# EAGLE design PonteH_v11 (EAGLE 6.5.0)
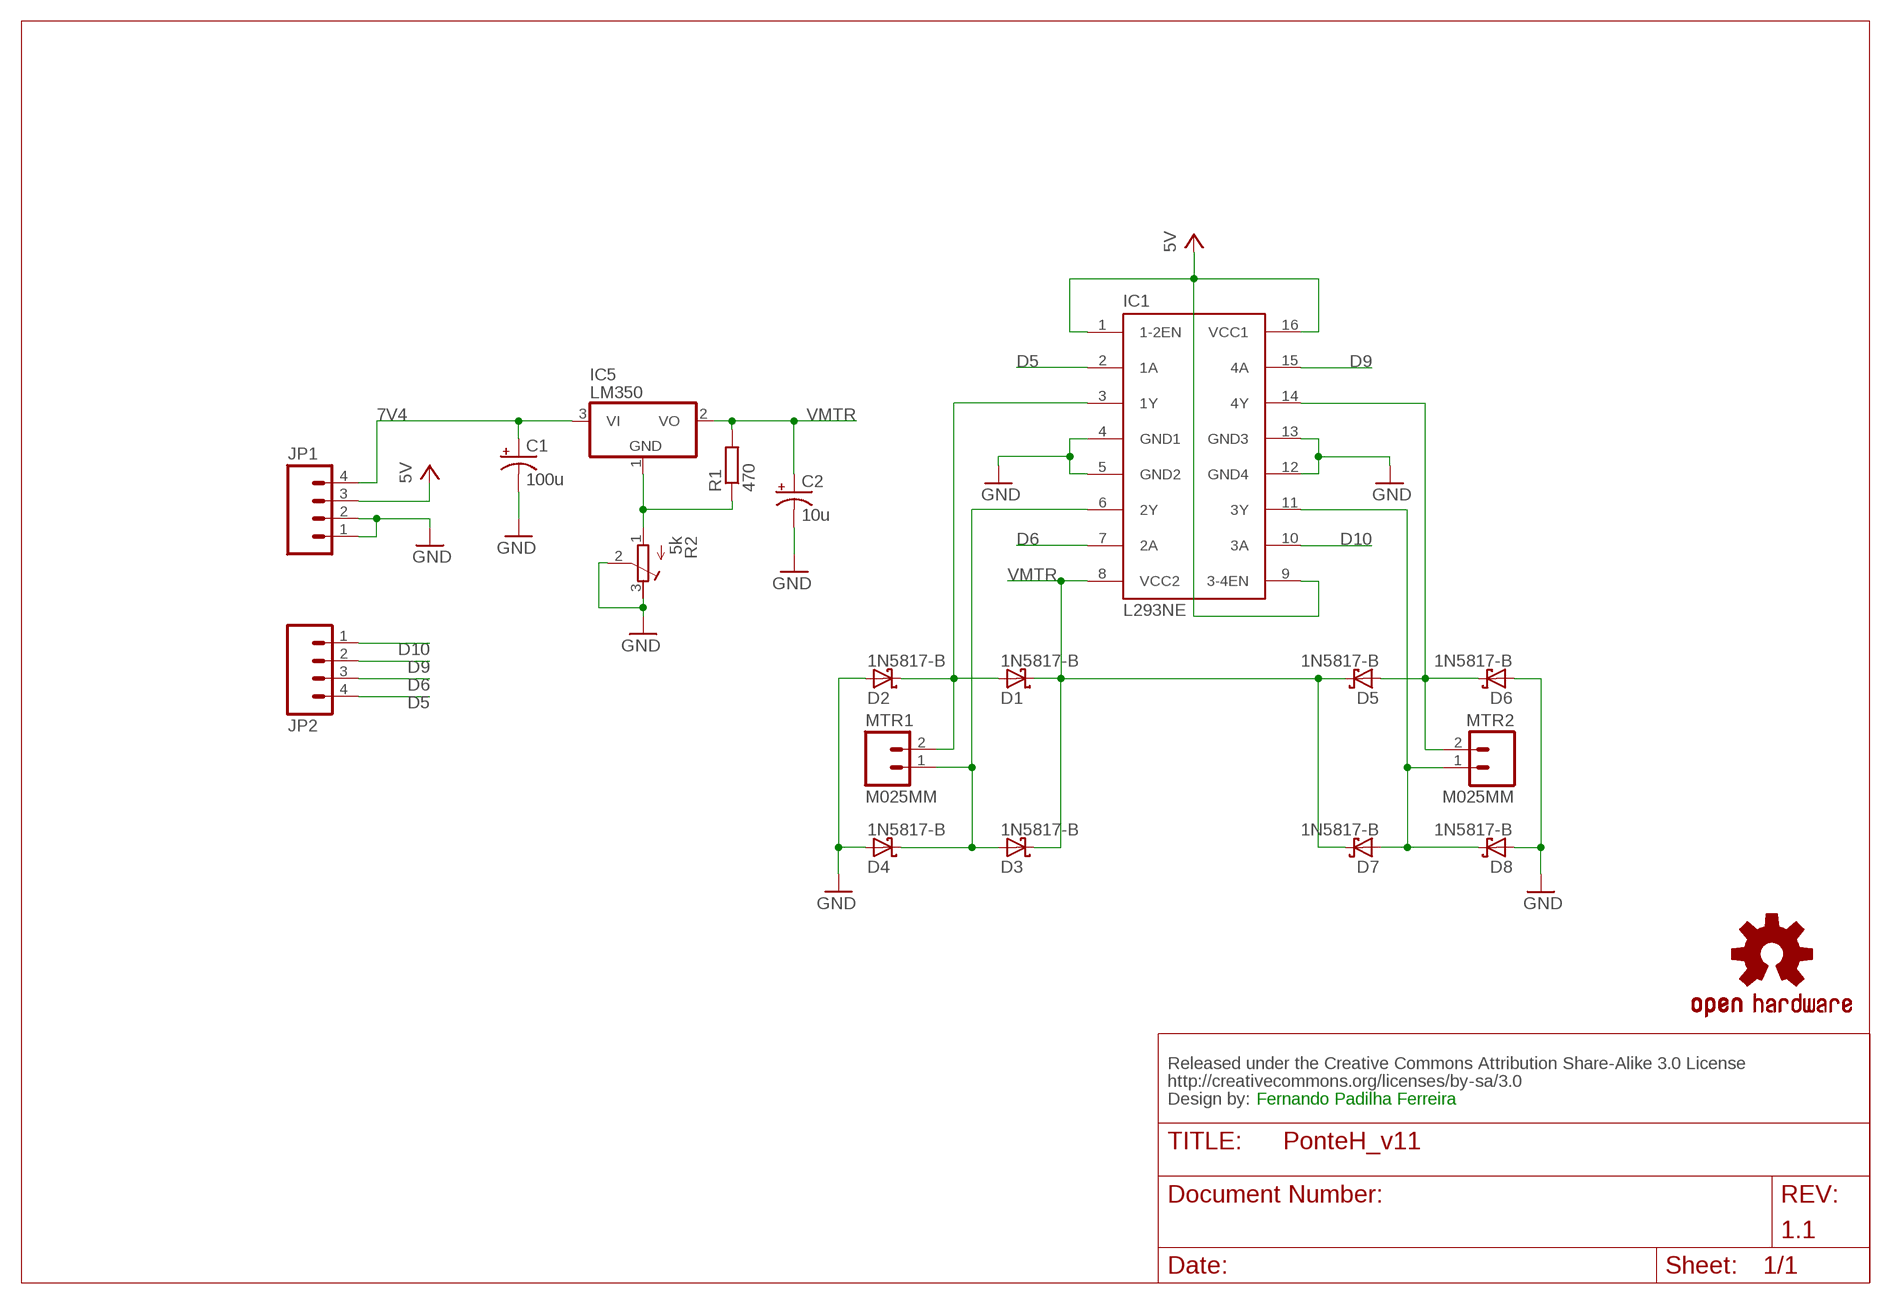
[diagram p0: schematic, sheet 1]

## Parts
C1  100u  CPOL-USE2.5-6  [E2,5-6]
C2  10u  CPOL-USE2.5-6  [E2,5-6]
CC_TEXT1  CREATIVE_COMMONS  [CREATIVE_COMMONS]
D1  1N5817-B  [DO41-7.6]
D2  1N5817-B  [DO41-7.6]
D3  1N5817-B  [DO41-7.6]
D4  1N5817-B  [DO41-7.6]
D5  1N5817-B  [DO41-7.6]
D6  1N5817-B  [DO41-7.6]
D7  1N5817-B  [DO41-7.6]
D8  1N5817-B  [DO41-7.6]
IC1  L293NE  L293E  [DIL16]
IC5  LM350  [TO220V]
JP1  M04PTH  [1X04]
JP2  M04PTH  [1X04]
LOGO1  OSHW-LOGOL  [OSHW-LOGO-L]
MTR1  M025MM  [SCREWTERMINAL-5MM-2]
MTR2  M025MM  [SCREWTERMINAL-5MM-2]
R1  470  R-EU_0207/7  [0207/7]
R2  5k  R-TRIMM64W  [RTRIM64W]

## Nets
5V [5v]: IC1.1(1-2EN) IC1.9(3-4EN) IC1.16(VCC1) JP1.3
7V4 [MTR]: C1.+ IC5.3(VI) JP1.4
D5 [SIGNAL]: IC1.2(1A) JP2.4
D6 [SIGNAL]: IC1.7(2A) JP2.3
D9 [SIGNAL]: IC1.15(4A) JP2.2
D10 [SIGNAL]: IC1.10(3A) JP2.1
GND: C1.- C2.- D2.A D4.A D6.A D8.A IC1.4(GND1) IC1.5(GND2) IC1.12(GND4) IC1.13(GND3) JP1.1 JP1.2 R2.2(S) R2.3(A)
M1A [MTR]: D1.A D2.C IC1.3(1Y) MTR1.2
M1B [MTR]: D3.A D4.C IC1.6(2Y) MTR1.1
M2A [MTR]: D5.A D6.C IC1.14(4Y) MTR2.2
M2B [MTR]: D7.A D8.C IC1.11(3Y) MTR2.1
N$1: IC5.1(GND) R1.1 R2.1(E)
VMTR [MTR]: C2.+ D1.C D3.C D5.C D7.C IC1.8(VCC2) IC5.2(VO) R1.2

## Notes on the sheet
- Fernando Padilha Ferreira
- 1.1

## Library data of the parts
C1 C2 = rcl:CPOL-US: POLARIZED CAPACITOR, American symbol
CC_TEXT1 = SparkFun-Aesthetics:CREATIVE_COMMONS: Creative Commons License summary
D1-D8 = diode:1N581*: 1.0A SCHOTTKY BARRIER RECTIFIER
IC1 = texas:L293E: TI DEVICE; MF: Arrow Electronics; MPN: L293E; OC_FARNELL: 1467711; OC_NEWARK: 89K0732
IC5 = linear:LM350: LM350 LM 350
JP1 JP2 = SparkFun-Connectors:M04: Header 4 Standard 4-pin 0.1" header. Use with straight break away headers (SKU : PRT-00116), right angle break away headers (PRT-00553), swiss pins (PRT-00743), machine pins (PRT-00117), and female headers (PRT-00115). Molex polarized connector foot print use with SKU : PRT-08231 with associated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
LOGO1 = SparkFun-Aesthetics:OSHW-LOGO: Open Source Hardware Logo This logo indicates the piece of hardware it is found on incorporates a OSHW license and/or adheres to the definition of open source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
MTR1 MTR2 = SparkFun-Connectors:M02: Standard 2-pin 0.1" header. Use with
R1 = resistor:R-EU_: RESISTOR, European symbol
R2 = resistor:R-TRIMM: Trimm resistor

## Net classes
0 GND: width 1.016 mm, clearance 0.406 mm
1 MTR: width 1.016 mm, clearance 0.406 mm
3 5v: width 0.508 mm

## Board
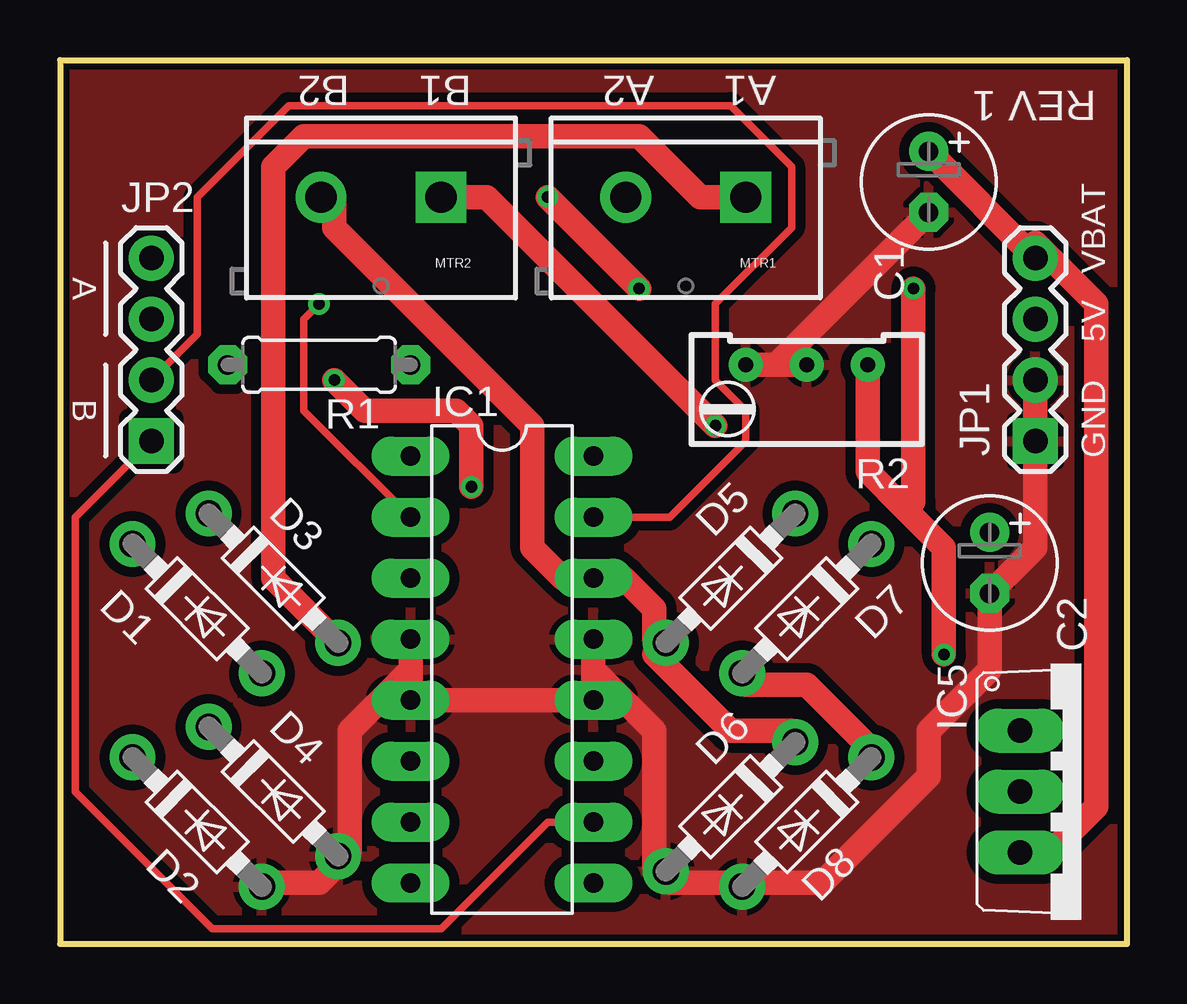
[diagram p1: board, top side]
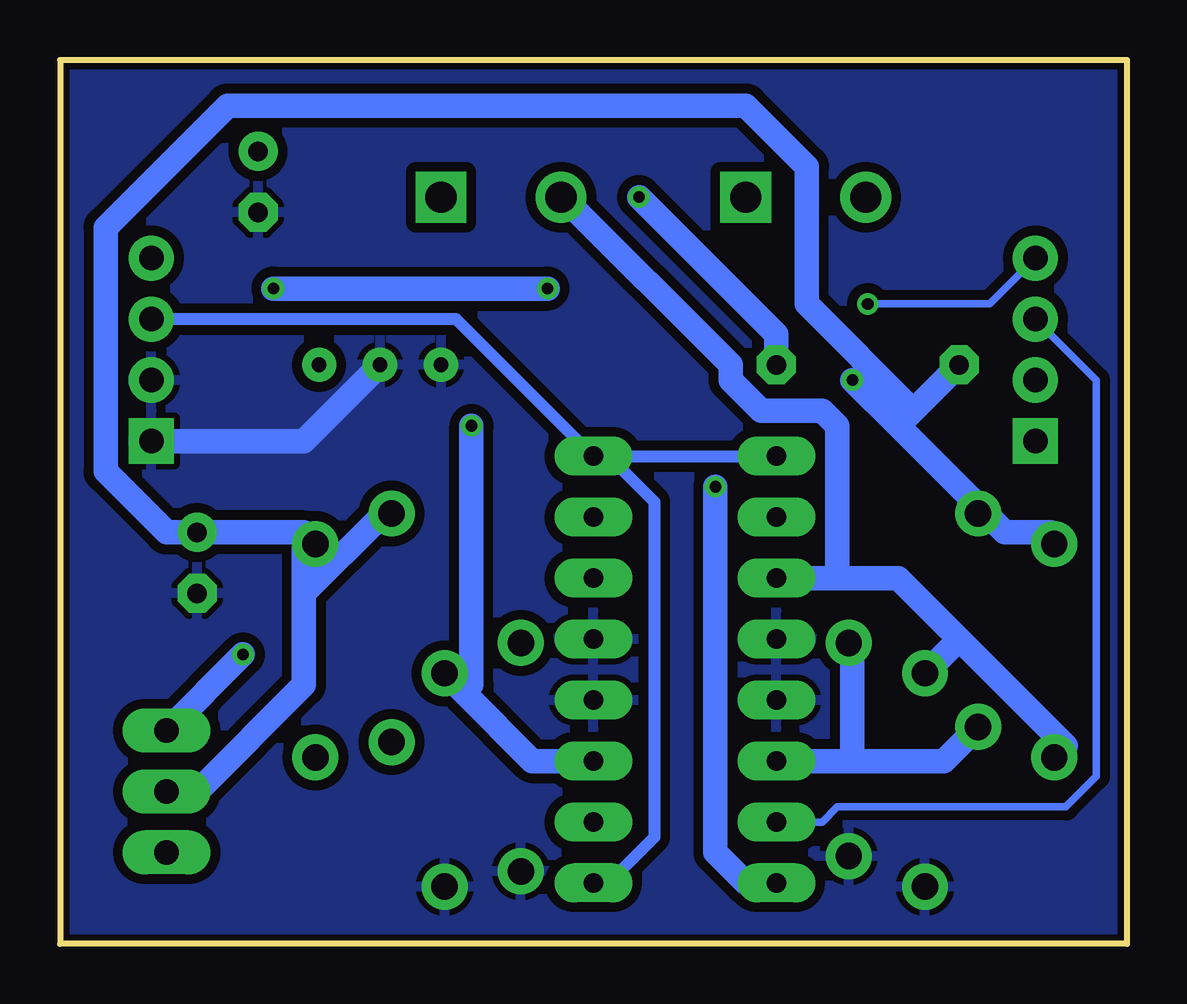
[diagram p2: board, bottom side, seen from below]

Size 44.45 x 36.83 mm. Coordinates in mm from the lower left corner, seen from the top.
Outline: 0,0 44.45,0 44.45,36.83 0,36.83 0,0
Copper layers (1*16): Top 0.035mm / dielectric 1.5mm / Bottom 0.035mm
Design rules "peteco": minimum track width 12mil, minimum drill 19mil, track to track 10mil, track to pad 10mil, pad to pad 10mil, via to via 10mil, smd to smd 0mil, copper to edge 10mil, drill to drill 8mil, minimum pad ring 16mil, minimum via ring 8mil, stop-mask expansion 4mil, vias tented up to drill 0mil, thermal gap 10mil

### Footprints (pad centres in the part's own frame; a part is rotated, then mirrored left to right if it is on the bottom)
E2,5-6 = drill 0.813 pad 1.6: + -1.27,0 | drill 0.813 pad 1.6 octagon: - 1.27,0
DO41-7.6 = drill 1.1 pad 1.7: A 3.81,0; C -3.81,0
DIL16 = drill 0.813 long: 1 -8.89,-3.81; 2 -6.35,-3.81; 3 -3.81,-3.81; 4 -1.27,-3.81; 5 1.27,-3.81; 6 3.81,-3.81; 7 6.35,-3.81; 8 8.89,-3.81; 9 8.89,3.81; 10 6.35,3.81; 11 3.81,3.81; 12 1.27,3.81; 13 -1.27,3.81; 14 -3.81,3.81; 15 -6.35,3.81; 16 -8.89,3.81
TO220V = drill 1.016 long: 1 -2.54,-2.54; 2 0,-2.54; 3 2.54,-2.54
1X04 = drill 1.016 pad 1.88 square: 1 0,0 | drill 1.016 pad 1.88: 2 2.54,0; 3 5.08,0; 4 7.62,0
SCREWTERMINAL-5MM-2 = drill 1.3 pad 2.032 square: 1 0,0 | drill 1.3 pad 2.032: 2 5,0
0207/7 = drill 0.813 octagon: 1 -3.81,0; 2 3.81,0
RTRIM64W = drill 0.61: 1 1.27,-2.54; 2 1.27,0; 3 1.27,2.54

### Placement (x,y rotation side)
C1  36.2,31.75 270 top
C2  38.73,15.88 270 top
CC_TEXT1  not placed on the board
D1  5.71,13.97 315 top
D2  5.71,5.08 315 top
D3  8.89,15.24 315 top
D4  8.89,6.35 315 top
D5  27.94,15.24 225 top
D6  27.94,5.71 225 top
D7  31.11,13.97 225 top
D8  31.11,5.08 225 top
IC1  18.41,11.43 270 top
IC5  42.55,6.35 270 top
JP1  40.64,20.95 90 top
JP2  3.81,20.95 90 top
LOGO1  not placed on the board
MTR1  28.57,31.11 180 top
MTR2  15.88,31.11 180 top
R1  10.79,24.13 180 top
R2  31.11,22.86 90 top

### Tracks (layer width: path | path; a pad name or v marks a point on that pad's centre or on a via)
5V
  Bottom 0.508: IC1.9 21.59,2.54 19.68,4.45 19.68,18.41 21.59,20.32 | 21.59,20.32 IC1.1 | 21.59,20.32 IC1.16 27.94,26.04 JP1.3
7V4
  Top 1.016: C1.+ JP1.4 40.64,29.21 43.18,26.67 43.18,5.71 41.27,3.81 IC5.3
D5  (via drill 0.48)
  Top 0.305: IC1.2 10.16,22.23 10.16,26.04 v10.79,26.67
  Bottom 0.305: v10.79,26.67 5.71,26.67 JP2.4
D6
  Bottom 0.305: IC1.7 12.7,5.08 12.06,5.71 2.54,5.71 1.27,6.99 1.27,23.5 JP2.3
D9
  Top 0.305: IC1.15 25.4,17.78 28.57,20.95 28.57,22.23 27.3,23.5 27.3,26.67 30.48,29.84 30.48,32.38 27.94,34.92 9.53,34.92 5.71,31.11 5.71,25.4 JP2.2
D10
  Top 0.305: IC1.10 20.32,5.08 15.88,0.64 6.35,0.64 0.64,6.35 0.64,17.78 JP2.1
GND
  Top 1.016: JP1.2 JP1.1 40.64,16.51 C2.- 38.73,11.43 36.2,8.89 36.2,6.99 31.75,2.54 28.57,2.54 D8.A 27.94,2.54 25.4,2.54 D6.A 24.77,3.17 24.77,8.89 22.23,11.43 | R2.2 29.84,24.13 | 29.84,24.13 R2.3 | 29.84,24.13 C1.- | D2.A 8.89,2.54 10.79,2.54 11.43,3.17 D4.A 12.06,3.81 12.06,8.89 14.61,11.43 | IC1.4 14.61,11.43 | 14.61,11.43 IC1.5 IC1.12 22.23,11.43 | IC1.13 22.23,11.43
  Bottom 1.016: JP1.1 34.29,20.95 R2.2
  pour Top: 0,0 44.45,0 44.45,36.83 0,36.83
  pour Bottom: 0,0 44.45,0 44.45,36.83 0,36.83
M1A
  Bottom 1.016: 12.06,15.24 9.53,15.24 6.99,12.7 | 12.06,15.24 IC1.3 | 6.99,12.7 2.54,8.26 D2.C | 6.99,12.7 8.26,11.43 D1.A | 12.06,15.24 12.06,21.59 12.7,22.23 15.24,22.23 16.51,23.5 16.51,24.13 23.5,31.11 MTR1.2
M1B
  Top 1.016: MTR1.1 26.67,31.11 24.13,33.66 10.16,33.66 8.89,32.38 8.89,15.24 11.43,12.7 D3.A
  Bottom 1.016: 11.43,7.62 7.62,7.62 6.35,8.89 D4.C | 11.43,7.62 IC1.6 | 11.43,7.62 11.43,12.06 D3.A
M2A
  Top 1.016: D6.C 30.48,8.89 27.94,8.89 24.77,12.06 D5.A 24.77,12.7 24.77,13.97 23.5,15.24 IC1.14 20.95,15.24 19.68,16.51 19.68,21.59 11.43,29.84 11.43,31.11 MTR2.2
M2B  (via drill 0.48)
  Top 1.016: D8.C 33.66,8.26 31.11,10.79 28.57,10.79 D7.A | MTR2.1 17.78,31.11 v27.3,21.59
  Bottom 1.016: IC1.11 24.77,7.62 27.62,10.48 | 27.62,10.48 D7.A | v27.3,21.59 27.3,10.79 27.62,10.48
N$1  (via drill 0.48)
  Top 1.016: R2.1 33.66,19.68 35.24,18.1 | 35.24,18.1 36.83,16.51 v36.83,12.06 | v24.13,27.3 v20.32,31.11 | v35.56,27.3 35.56,18.41 35.24,18.1
  Bottom 1.016: IC5.1 v36.83,12.06 | R1.1 14.61,25.4 v20.32,31.11 | v35.56,27.3 v24.13,27.3
VMTR  (via drill 0.48)
  Top 1.016: v17.14,19.05 17.14,21.59 16.51,22.23 12.7,22.23 v11.43,23.5
  Bottom 1.016: IC5.2 38.73,6.35 34.29,10.79 34.29,14.61 | 34.29,14.61 34.29,16.51 D7.C 34.29,17.14 C2.+ 40.01,17.14 42.55,19.68 42.55,29.84 37.47,34.92 15.88,34.92 13.34,32.38 13.34,26.67 8.89,22.23 | 34.29,14.61 31.11,17.78 D5.C | IC1.8 15.88,2.54 17.14,3.81 v17.14,19.05 | 9.53,21.59 6.35,18.41 D3.C 5.71,17.78 5.08,17.14 3.17,17.14 D1.C | 9.53,21.59 v11.43,23.5 | 9.53,21.59 8.89,22.23 | 8.89,22.23 R1.2

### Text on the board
tPlace: B2 | B1 | A2 | A1 | REV 1 | VBAT | A | 5V | GND | B
tDocu: Fernando Padilha Ferreira

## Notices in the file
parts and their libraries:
SparkFun-Connectors: Licensing: CC v3.0 Share-Alike You are welcome to use this library for commercial purposes.
SparkFun-Aesthetics: Released under the Creative Commons Attribution Share-Alike 3.0 License
SparkFun-Aesthetics: http://creativecommons.org/licenses/by-sa/3.0
